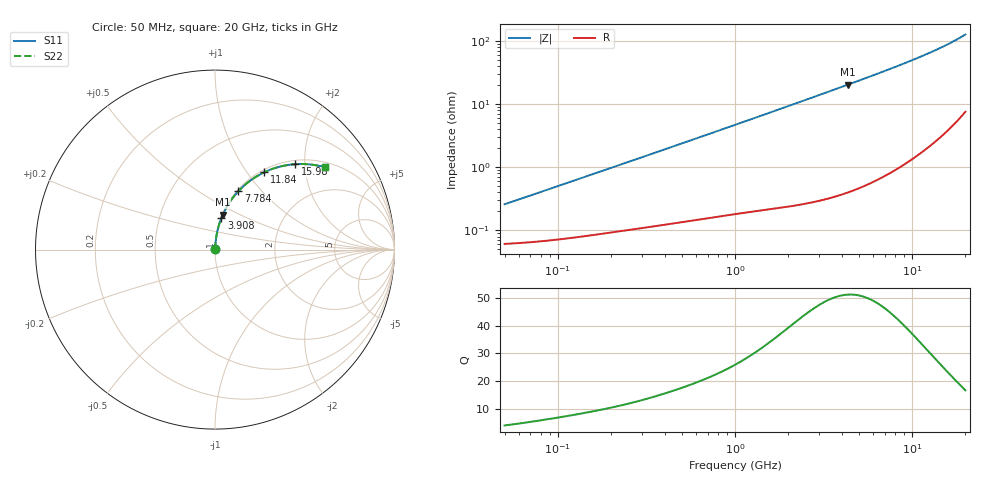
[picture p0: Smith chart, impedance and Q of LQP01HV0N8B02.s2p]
!Murata Part Number: LQP01HV0N8B02
!These Parameters are Measured in Series Mode Connection
!  o--[Z]--o
!Port1  Port2
!  o-------o
!Freq. Start=50[MHz] Stop=20[GHz], 401[Steps]
# Hz S RI R 50
!Freq.(Hz) S11(Real) S11(Imag) S21(Real) S21(Imag) S12(Real) S12(Imag) S22(Real) S22(Imag)
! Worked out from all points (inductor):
!   401 points, 50 MHz to 20 GHz, reference 50 ohm
!   read as one part in series: L = 800 pH near 51.52 MHz
!   highest Q = 51.1 at 4.34 GHz (marker M1), where L = 747 pH
!   S11 on the Smith chart (normalised r, x): 50 MHz: 1.00, +0.01; 3.908 GHz: 1.01, +0.37; 7.784 GHz: 1.02, +0.75; 11.84 GHz: 1.04, +1.21; 15.98 GHz: 1.08, +1.79; 20 GHz: 1.15, +2.54
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5e7  0.000616 0.00252  0.9994 -0.00252  0.9994 -0.00252  0.000616 0.00252
5.552724e7  0.000628 0.00279  0.9994 -0.00279  0.9994 -0.00279  0.000628 0.00279
1.364002e8  0.000842 0.00672  0.9992 -0.00672  0.9992 -0.00672  0.000842 0.00672
3.721004e8  0.00151 0.0178  0.9985 -0.0178  0.9985 -0.0178  0.00151 0.0178
6.380365e8  0.0024 0.0301  0.9976 -0.0301  0.9976 -0.0301  0.0024 0.0301
1e9  0.00399 0.0466  0.996 -0.0466  0.996 -0.0466  0.00399 0.0466
1.714689e9  0.00853 0.0791  0.9915 -0.0791  0.9915 -0.0791  0.00853 0.0791
2.728004e9  0.0186 0.1245  0.9814 -0.1245  0.9814 -0.1245  0.0186 0.1245
3.908127e9  0.0356 0.1758  0.9644 -0.1758  0.9644 -0.1758  0.0356 0.1758
4.34015e9  0.0433 0.194  0.9567 -0.194  0.9567 -0.194  0.0433 0.194
5.769027e9  0.0739 0.2517  0.9261 -0.2517  0.9261 -0.2517  0.0739 0.2517
7.442007e9  0.119 0.3128  0.881 -0.3128  0.881 -0.3128  0.119 0.3128
7.784049e9  0.1293 0.3244  0.8707 -0.3244  0.8707 -0.3244  0.1293 0.3244
8.774992e9  0.1612 0.3557  0.8388 -0.3557  0.8388 -0.3557  0.1612 0.3557
9.745021e9  0.195 0.3832  0.805 -0.3832  0.805 -0.3832  0.195 0.3832
1.082228e10  0.235 0.4098  0.765 -0.4098  0.765 -0.4098  0.235 0.4098
1.183995e10  0.2747 0.431  0.7253 -0.431  0.7253 -0.431  0.2747 0.431
1.375312e10  0.3531 0.4601  0.6469 -0.4601  0.6469 -0.4601  0.3531 0.4601
1.597544e10  0.4469 0.476  0.5531 -0.476  0.5531 -0.476  0.4469 0.476
1.774144e10  0.5209 0.4753  0.4791 -0.4753  0.4791 -0.4753  0.5209 0.4753
1.940974e10  0.5884 0.4645  0.4116 -0.4645  0.4116 -0.4645  0.5884 0.4645
2e10  0.6114 0.4585  0.3886 -0.4585  0.3886 -0.4585  0.6114 0.4585
